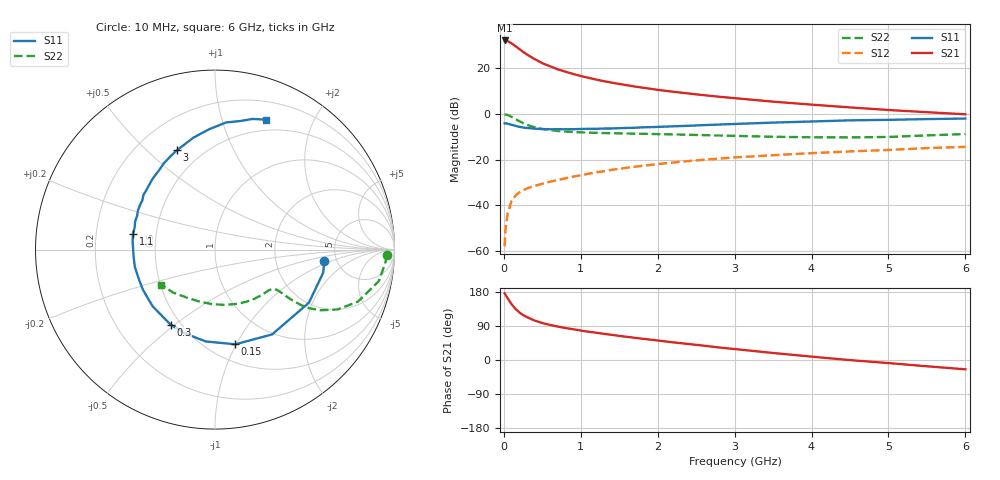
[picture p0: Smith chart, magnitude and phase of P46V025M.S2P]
! SIEMENS Small Signal Semiconductors
! BFP182
! Si NPN RF Bipolar Junction Transistor in SOT143
! VCE = 6 V  IC = 25 mA
! Common Emitter S-Parameters:  March  1996
# GHz  S  MA  R  50
!  f  S11  S21  S12  S22
! GHz  MAG  ANG  MAG  ANG  MAG  ANG  MAG  ANG
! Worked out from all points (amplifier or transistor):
!   36 points, 10 MHz to 6 GHz, reference 50 ohm
!   highest |S21| = 31.8 dB at 10 MHz (marker M1)
!   |S21| within 3 dB of that: start of sweep to 171.6 MHz
!   unconditionally stable (mu >= 1): 750.1 MHz to 5.424 GHz
!   at 250 MHz: K = 0.52, MSG = 30.2 dB, |S12| = -33.5 dB
!   at 1.4 GHz: K = 1.15, MAG = 16.6 dB, |S12| = -24.5 dB
!   at 6 GHz: K = 0.95, MSG = 7.1 dB, |S12| = -14.5 dB
!   S11 on the Smith chart (normalised r, x): 10 MHz: 3.99, -0.79; 150 MHz: 0.67, -0.99; 300 MHz: 0.44, -0.48; 1.1 GHz: 0.37, +0.08; 3 GHz: 0.37, +0.62; 6 GHz: 0.38, +1.40
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0.01  0.6122 -5.8  38.95 175.9  0.0013 80.3  0.9574 -1.8
0.02  0.6163 -12.1  38.84 172.9  0.0029 83.3  0.9527 -4.2
0.05  0.601 -29.5  37.68 162.5  0.0067 81.5  0.9296 -10.9
0.1  0.5697 -56.1  33.66 147.4  0.0125 65.6  0.8476 -20.0
0.15  0.5396 -77.9  29.35 135.2  0.0163 60.2  0.7607 -26.0
0.2  0.5143 -95.7  25.41 125.8  0.0192 55.4  0.682 -29.7
0.25  0.4965 -109.0  21.98 118.5  0.0212 53.1  0.6185 -31.9
0.3  0.4856 -120.7  19.32 113.1  0.0235 51.9  0.5689 -32.8
0.4  0.4696 -137.6  15.32 104.1  0.0266 52.2  0.5027 -33.3
0.5  0.4598 -150.8  12.52 97.6  0.0296 51.3  0.4616 -33.1
0.6  0.455 -159.6  10.69 92.6  0.0328 52.7  0.4356 -33.0
0.7  0.4567 -167.8  9.187 88.3  0.0357 53.4  0.4178 -33.0
0.8  0.4552 -175.0  8.152 84.4  0.0389 54.5  0.4062 -33.2
1  0.4615 174.0  6.548 77.7  0.0454 54.6  0.3899 -34.2
1.1  0.4655 169.2  5.993 74.6  0.0489 55.1  0.3846 -35.1
1.5  0.4805 153.6  4.405 63.6  0.0628 53.8  0.3707 -39.6
2.2  0.5271 130.9  2.984 46.6  0.0861 49.6  0.3518 -51.0
3  0.5929 111.0  2.162 28.9  0.111 42.6  0.327 -67.7
3.5  0.6352 100.9  1.816 18.5  0.124 38.0  0.3125 -80.0
4.5  0.711 85.0  1.359 -0.3  0.15 29.4  0.3021 -107.3
5.5  0.7573 74.0  1.07 -16.6  0.1773 21.3  0.3344 -134.3
6  0.7783 68.5  0.962 -24.5  0.1884 16.5  0.3582 -147.1
